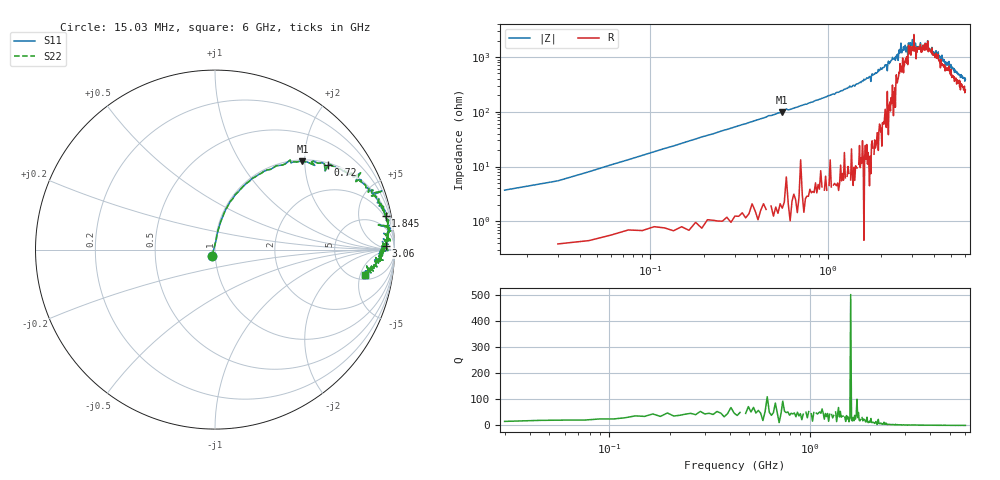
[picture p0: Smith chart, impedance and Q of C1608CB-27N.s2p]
!	Network	Analyzer	HP8753E.07.74:	Oct	30	2002	Serial	No.	JP38451487
!	Hewlett-Packard
!	7	Sep	2009	9:41:10
!	Frequency	S11	S21	S12	S22
#	HZ	S	RI	R	50
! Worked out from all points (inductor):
!   400 points, 15.03 MHz to 6 GHz, reference 50 ohm
!   read as one part in series: L = 28.4 nH near 45.03 MHz
!   highest Q = 51.8 at 555 MHz (marker M1), where L = 27.9 nH
!   self-resonance near 3.06 GHz
!   S11 on the Smith chart (normalised r, x): 15.03 MHz: 0.97, -0.06; 720 MHz: 1.06, +2.63; 1.845 GHz: 2, +10; 3.06 GHz: 33, +15; 6 GHz: 6.01, -6.03
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1.502992e7  -0.0161 -0.0332  1.02 0.0332  1.02 0.0332  -0.0161 -0.0332
7.502962e7  0.0239 0.129  0.976 -0.129  0.976 -0.129  0.0239 0.129
1.650292e8  0.0841 0.266  0.916 -0.266  0.916 -0.266  0.0841 0.266
5.550272e8  0.487 0.491  0.513 -0.491  0.513 -0.491  0.487 0.491
7.200264e8  0.631 0.471  0.369 -0.471  0.369 -0.471  0.631 0.471
1.020025e9  0.79 0.396  0.21 -0.396  0.21 -0.396  0.79 0.396
1.845021e9  0.951 0.187  0.0488 -0.187  0.0488 -0.187  0.951 0.187
2.01002e9  0.961 0.157  0.0393 -0.157  0.0393 -0.157  0.961 0.157
2.505017e9  0.94 0.0908  0.0602 -0.0908  0.0602 -0.0908  0.94 0.0908
2.595017e9  0.977 0.0492  0.0232 -0.0492  0.0232 -0.0492  0.977 0.0492
2.625017e9  0.959 0.0694  0.0409 -0.0694  0.0409 -0.0694  0.959 0.0694
2.835016e9  0.938 0.0606  0.0615 -0.0606  0.0615 -0.0606  0.938 0.0606
2.865016e9  0.952 0.0208  0.0483 -0.0208  0.0483 -0.0208  0.952 0.0208
3.015015e9  0.965 0.0301  0.0352 -0.0301  0.0352 -0.0301  0.965 0.0301
3.060015e9  0.951 0.022  0.0495 -0.022  0.0495 -0.022  0.951 0.022
3.075015e9  0.963 -0.00565  0.0369 0.00565  0.0369 0.00565  0.963 -0.00565
3.165014e9  0.933 0.0453  0.0667 -0.0453  0.0667 -0.0453  0.933 0.0453
3.675012e9  0.953 -0.00702  0.0474 0.00702  0.0474 0.00702  0.953 -0.00702
3.705011e9  0.926 -0.00354  0.0736 0.00354  0.0736 0.00354  0.926 -0.00354
4.00501e9  0.932 -0.0341  0.0685 0.0341  0.0685 0.0341  0.932 -0.0341
5.010005e9  0.895 -0.083  0.105 0.083  0.105 0.083  0.895 -0.083
6e9  0.836 -0.141  0.164 0.141  0.164 0.141  0.836 -0.141
